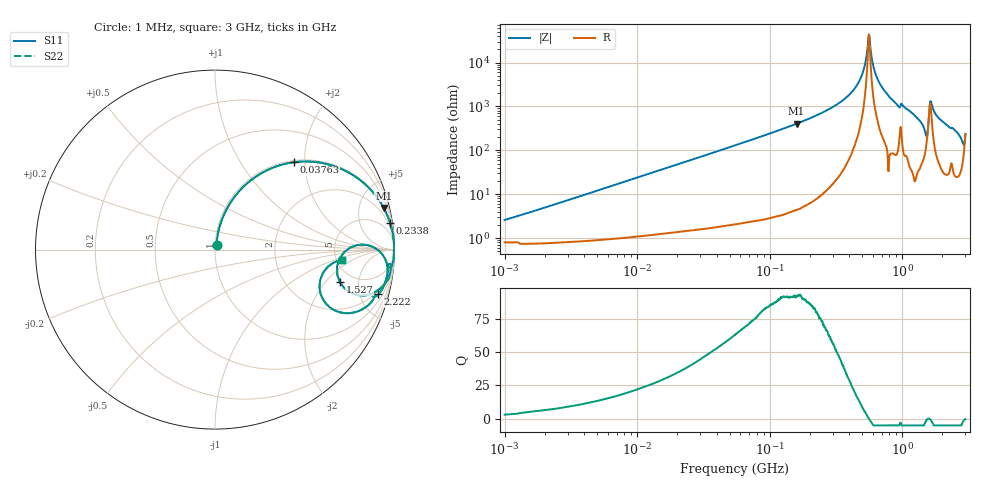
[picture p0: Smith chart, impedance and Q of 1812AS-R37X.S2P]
!s-Parameter Generated by FASTRON Sdn. Bhd.
!FASTRON P/N : 1812AS-R37X
!Keysight Technologies,E4991B,MY54100416,A.01.15
!Date created: Fri Oct 13 15:12:48 2023
!Version  : Rev00 Fri Oct 13 15:12:48 2023
!Data & Calibration Information:
!Freq	S11	S21	S12	S22
!PortZ  Port1:50+j0  Port2:50+j0
!When reading, reference impedance value at option line is always used.
! Remarks : This data is being provided solely for informational purposes.
# Hz S dB R 50
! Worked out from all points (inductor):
!   1601 points, 1 MHz to 3 GHz, reference 50 ohm
!   read as one part in series: L = 391 nH near 1.041 MHz
!   highest Q = 91.9 at 159.8 MHz (marker M1), where L = 403 nH
!   self-resonance near 561.2 MHz
!   S11 on the Smith chart (normalised r, x): 1 MHz: 1.02, +0.05; 37.63 MHz: 1.03, +1.77; 233.8 MHz: 1, +13; 1.527 GHz: 3.85, -2.89; 2.222 GHz: 1.56, -7.09; 3 GHz: 5.54, -1.26
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1000000  -31.81 70.6  -0.07 -1.4  -0.07 -1.4  -31.81 70.6
3804036  -20.82 79.5  -0.11 -5.2  -0.11 -5.2  -20.82 79.5
1.447069e7  -9.88 69.3  -0.58 -18.7  -0.58 -18.7  -9.88 69.3
3.763315e7  -3.65 47.8  -2.60 -41.1  -2.60 -41.1  -3.65 47.8
5.477226e7  -2.10 37.4  -4.34 -51.7  -4.34 -51.7  -2.10 37.4
1.59818e8  -0.28 13.9  -12.41 -75.5  -12.41 -75.5  -0.28 13.9
2.083556e8  -0.15 10.1  -15.13 -79.2  -15.13 -79.2  -0.15 10.1
2.3377e8  -0.12 8.7  -16.45 -80.6  -16.45 -80.6  -0.12 8.7
3.436571e8  -0.04 4.5  -22.10 -84.2  -22.10 -84.2  -0.04 4.5
4.391493e8  -0.02 2.2  -28.27 -84.9  -28.27 -84.9  -0.02 2.2
5.026765e8  -0.02 1.0  -35.14 -82.1  -35.14 -82.1  -0.02 1.0
5.611759e8  -0.02 0.0  -52.79 -4.5  -52.79 -4.5  -0.02 0.0
6.423554e8  -0.02 -1.2  -33.39 81.8  -33.39 81.8  -0.02 -1.2
7.925923e8  -0.03 -3.3  -24.67 85.2  -24.67 85.2  -0.03 -3.3
1.307284e9  -0.24 -10.5  -14.78 76.1  -14.78 76.1  -0.24 -10.5
1.45942e9  -0.86 -15.8  -11.13 62.5  -11.13 62.5  -0.86 -15.8
1.526649e9  -2.87 -14.6  -9.02 30.8  -9.02 30.8  -2.87 -14.6
1.662201e9  -0.39 -3.9  -21.91 54.4  -21.91 54.4  -0.39 -3.9
1.846379e9  -0.28 -9.5  -15.59 74.4  -15.59 74.4  -0.28 -9.5
2.221924e9  -0.51 -15.3  -11.52 70.1  -11.52 70.1  -0.51 -15.3
2.769173e9  -1.60 -25.2  -7.30 55.1  -7.30 55.1  -1.60 -25.2
3e9  -3.01 -4.6  -10.45 11.0  -10.45 11.0  -3.01 -4.6
